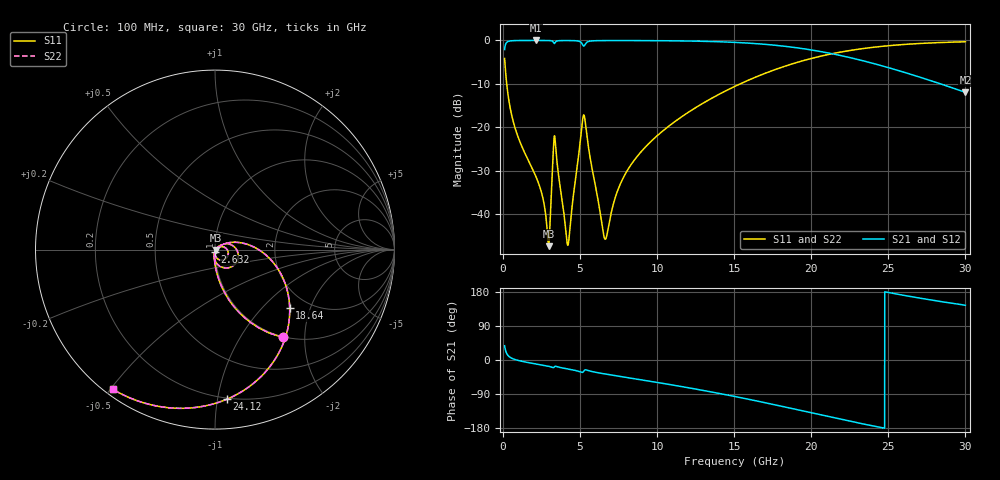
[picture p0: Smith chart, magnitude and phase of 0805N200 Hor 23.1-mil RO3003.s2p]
# GHz S MA R 50
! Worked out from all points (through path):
!   3201 points, 100 MHz to 30 GHz, reference 50 ohm
!   highest |S21| = -0.02 dB at 2.128 GHz (marker M1); lowest = -12.0 dB at 30 GHz (marker M2)
!   group delay of S21, straight-line fit = 21.2 ps
!   lowest |S11| = -47.4 dB at 2.959 GHz (marker M3), VSWR 1.01, Z = 50.4 - j0.21 ohm
!   |S11| at or under -10 dB: 236 MHz to 15.39 GHz (15.15 GHz wide, 194 % of centre)
!   |S22| runs from -47.4 to -0.3 dB; largest |S21 - S12| = 0
!   S11 on the Smith chart (normalised r, x): 100 MHz: 0.99, -1.56; 2.632 GHz: 1.00, -0.03; 18.64 GHz: 1.61, -1.46; 24.12 GHz: 0.19, -1.06; 30 GHz: 0.02, -0.51
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0.1  0.619 -52.3  0.785 37.7  0.785 37.7  0.619 -52.3
0.3335938  0.229 -78.5  0.9728 11.3  0.9728 11.3  0.229 -78.5
0.7260313  0.1056 -87.6  0.9935 1.9  0.9935 1.9  0.1056 -87.6
2.127594  0.0272 -97.2  0.998 -10.5  0.998 -10.5  0.0272 -97.2
2.632156  0.01397 -95.1  0.9976 -14.1  0.9976 -14.1  0.01397 -95.1
2.959188  0.00429 -29.1  0.9957 -16.7  0.9957 -16.7  0.00429 -29.1
3.061969  0.009207 25.8  0.9932 -17.7  0.9932 -17.7  0.009207 25.8
3.248844  0.04877 18.4  0.9613 -20.1  0.9613 -20.1  0.04877 18.4
3.370312  0.07373 -51.3  0.9384 -16.6  0.9384 -16.6  0.07373 -51.3
4.089781  0.00595 -66.9  0.9956 -22.8  0.9956 -22.8  0.00595 -66.9
4.239281  0.004598 -9.7  0.9954 -23.9  0.9954 -23.9  0.004598 -9.7
5.089563  0.09423 16.3  0.9354 -32.6  0.9354 -32.6  0.09423 16.3
5.323156  0.1189 -59.6  0.8985 -26.1  0.8985 -26.1  0.1189 -59.6
6.631281  0.005147 -31.9  0.9946 -36.9  0.9946 -36.9  0.005147 -31.9
7.836625  0.02704 36.2  0.9952 -44.9  0.9952 -44.9  0.02704 36.2
10.06978  0.082 27.3  0.9918 -59.6  0.9918 -59.6  0.082 27.3
15.05  0.2964 -7.6  0.9482 -96.4  0.9482 -96.4  0.2964 -7.6
18.638  0.5283 -38.0  0.8405 -127.1  0.8405 -127.1  0.5283 -38.0
20.03956  0.6217 -50.5  0.774 -139.7  0.774 -139.7  0.6217 -50.5
24.12278  0.8368 -85.6  0.5368 -174.9  0.5368 -174.9  0.8368 -85.6
25.01978  0.8685 -92.6  0.4849 178.0  0.4849 178.0  0.8685 -92.6
30  0.9641 -126.1  0.2525 144.5  0.2525 144.5  0.9641 -126.1
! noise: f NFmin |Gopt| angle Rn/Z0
0.1  0.000554  0.8899  0.8764  0.001095
3.417  0.02643  0.9204  19.3  0.07132
6.743  0.01365  0.7316  37.51  0.009116
10.06  0.01576  0.6749  54.49  0.007464
13.39  0.02028  0.6753  70.32  0.008205
16.7  0.02594  0.6916  84.94  0.009163
20.03  0.03327  0.7183  98.64  0.01029
23.35  0.0432  0.7529  111.6  0.01162
26.67  0.05752  0.7942  124.3  0.0132
30  0.07951  0.8391  136.8  0.01486
